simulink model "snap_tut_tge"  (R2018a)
settings: Solver=VariableStepDiscrete  StartTime=0.0  StopTime=50000  RelTol=1e-3
undefined symbols (not defined in the file): bad_frame, Bit, Both, bram, c, cnt_rst, core_rst, d, data, data_in, eof, eof_in, Falling, hex2dec, ip, ip_in, led, led_rx, led_tx, led_up, link_up, Location, Lower, Minimum_Area, notused, out, overrun, reg, Rising, ROACH2, sfp, SNAP, tx_full, tx_over, Unsigned, Upper, valid, valid_in, Width, xc7k160t
libraries: xbsIndex_r4 x1201, casper_library_misc x9, xps_library x5
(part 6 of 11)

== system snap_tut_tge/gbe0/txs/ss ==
  note: Generate stop when in circular capture mode
  note: Delay start of capture
  note: ctrl: bit0: Put a posedge here to enable a new capture. bit1: ignore external trigger and trigger immediately. bit2: ignore external write enable and capture on every FPGA clock. bit3: continuously capture data until we get an external stop command.
  note: Offset in vector from first element captured, used during circular capture
  note: Number of bytes in buffer and done bit
  note: Number of valid data samples to skip after trigger before starting capture
  note: Value on vin aligned with first sample on din captured
  din : Inport
  we : Inport  Port=2
  trig : Inport  Port=3
  add_del : xbsIndex_r4/Delay  rst=off  infoeditControl=Selection of Reset will increase slice count due to use of real FFs and instead of SRLs  en=off  latency=1  reg_retiming=on  dbl_ovrd=off  block_type=delay
  add_gen : Subsystem  AncestorBlock=casper_library_scopes/snapshot/add_gen  mask{counter_size=13+4+1, increment=16, nsamples=13, burst_size=0, use_dsp48=on}
      mask prompts: counter_size "Address counter size (2^?)"; increment "Address counter increment"; nsamples "Number of samples (2^?)"; burst_size "Burst size (2^?)"; use_dsp48 "dsp48 counter/s"
      mask init:
      | set_param(gcb,'LinkStatus','inactive');
      | if strcmp(use_dsp48,'on'),
      |     set_param([gcb,'/add_gen'],'implementation','DSP48');
      | else
      |     set_param([gcb,'/add_gen'],'implementation','Fabric');
      | end
  arm : xbsIndex_r4/Constant  const=0  gui_display_data_type=Fixed-point  arith_type=Boolean  n_bits=16  bin_pt=14  preci_type=Single  exp_width=8  frac_width=24  explicit_period=on  period=1  equ=P=C  opselect=C  inp2=PCIN>>17  opr=+  inp1=P  carry=CIN  dbl_ovrd=off  block_type=constant
  arm_or : xbsIndex_r4/Logical  logical_function=OR  inputs=2  en=off  latency=0  precision=Full  arith_type=Unsigned  n_bits=16  bin_pt=0  align_bp=on  dbl_ovrd=off  block_type=logical
  basic_ctrl : Subsystem  AncestorBlock=casper_library_scopes/snapshot/basic_ctrl  mask{dram=off, data_width=128}
      mask prompts: data_width "data width"
      mask init:
      | set_param(gcb,'LinkStatus','inactive');
      | set_param([gcb,'/dram_munge'], 'dram', dram);
  bram : Subsystem  Tag=xps:bram  AncestorBlock=xps_library/Memory/shared_bram  mask{arith_type=Unsigned, addr_width=13, data_width=128, reg_prim_output=off, reg_core_output=off, optimization=Minimum_Area, data_bin_pt=0, init_vals=[0:2^13-1], sample_rate=1}
      mask prompts: arith_type "Output Data Type"; addr_width "Address width"; data_width "Data Width"; reg_prim_output "Register Primitive Output"; reg_core_output "Register Core Output"; data_bin_pt "Data Binary Point"; init_vals "Initial values (simulation only)"; sample_rate "Sample rate"
      mask init:
      | shared_bram_mask;
  cast : xbsIndex_r4/Convert  gui_display_data_type=Fixed-point  arith_type=Unsigned  n_bits=128  bin_pt=0  float_type=Single  exp_bits=8  fraction_bits=24  quantization=Truncate  overflow=Wrap  en=off  latency=0  pipeline=off  dbl_ovrd=off  block_type=convert
  circ : xbsIndex_r4/Constant  const=0  gui_display_data_type=Fixed-point  arith_type=Boolean  n_bits=16  bin_pt=14  preci_type=Single  exp_width=8  frac_width=24  explicit_period=on  period=1  equ=P=C  opselect=C  inp2=PCIN>>17  opr=+  inp1=P  carry=CIN  dbl_ovrd=off  block_type=constant
  circ_or : xbsIndex_r4/Logical  logical_function=OR  inputs=2  en=off  latency=0  precision=Full  arith_type=Unsigned  n_bits=16  bin_pt=0  align_bp=on  dbl_ovrd=off  block_type=logical
  ctrl : Subsystem  Tag=xps:sw_reg  AncestorBlock=xps_library/Memory/software_register  mask(swreg){io_dir=From Processor, io_delay=0, init_val=0, sample_period=1, names=reg, bitwidths=32, bin_pts=0, arith_types=0, sim_port=off, show_format=on}
      mask prompts: io_dir "I/O direction"; io_delay "I/O delay"; init_val "Initial Value"; sample_period "Sample period"; names "Bitfield names [msb...lsb]"; bitwidths "Bitfield widths"; bin_pts "Bitfield binary pts"; arith_types "Bitfield types, ufix=0, fix=1, bool=2"; sim_port "Provide sim input/output?"; show_format "Print format string?"
      mask help: A 32-bit software-accessible register. Can be divided into bitfields of varying widths and types using the fields in the block mask.
      mask init:
      | swreg_init(gcb)
  ctrl_combine : Subsystem  AncestorBlock=casper_library_flow_control/bus_create  mask(bus_create){inputNum=4}
      mask prompts: inputNum "Number of inputs:"
      mask init:
      | bus_create_init(gcb,...
      |     'inputNum', inputNum);
  ctrl_split : Subsystem  AncestorBlock=casper_library_flow_control/bus_expand  mask(bus_expand){mode=divisions of arbitrary size, outputNum=1, outputWidth=[28 1 2 1], outputBinaryPt=0, outputArithmeticType=[0 2 0 2], show_format=on, outputToWorkspace=off, variablePrefix=out, outputToModelAsWell=on}
      mask prompts: outputNum "Number of outputs:"; outputWidth "Output width [msb ... lsb]:"; outputBinaryPt "Output binary point position [msb ... lsb]:"; outputArithmeticType "Output arithmetic type (ufix=0, fix=1, bool=2) [msb ... lsb]:"; show_format "Print format string?"; outputToWorkspace "Output to workspace?"; variablePrefix "Variable name prefix:"; outputToModelAsWell "Output to model as well?"
      mask help: Expands a 'bus' made using a bus_create or Xilinx concat block. The input will be divided into the specified number of outputs with the specified arithmetic types. Divisions are made from most significant bit.
      mask init:
      | bus_expand_init(gcb,...
      |     'mode', mode, ...
      |     'outputNum', outputNum, ...
      |     'outputWidth', outputWidth, ...
      |     'outputBinaryPt', outputBinaryPt, ...
      |     'outputArithmeticType', outputArithmeticType, ...
      |     'show_format', show_format, ...
      |     'outputToWorkspace', outputToWorkspace, ...
      |     'variablePrefix', variablePrefix, ...
      |     'outputToModelAsWell', outputToModelAsWell);
  dat_del : xbsIndex_r4/Delay  rst=off  infoeditControl=Selection of Reset will increase slice count due to use of real FFs and instead of SRLs  en=off  latency=1  reg_retiming=on  dbl_ovrd=off  block_type=delay
  g_tr_en_cnt : Terminator
  gbram : Terminator
  goto_ss_we2_const : xbsIndex_r4/Constant  const=0  gui_display_data_type=Fixed-point  arith_type=Boolean  n_bits=16  bin_pt=14  preci_type=Single  exp_width=8  frac_width=24  explicit_period=on  period=1  equ=P=C  opselect=C  inp2=PCIN>>17  opr=+  inp1=P  carry=CIN  dbl_ovrd=off  block_type=constant
  goto_ss_we3_const : xbsIndex_r4/Constant  const=0  gui_display_data_type=Fixed-point  arith_type=Boolean  n_bits=16  bin_pt=14  preci_type=Single  exp_width=8  frac_width=24  explicit_period=on  period=1  equ=P=C  opselect=C  inp2=PCIN>>17  opr=+  inp1=P  carry=CIN  dbl_ovrd=off  block_type=constant
  gval : Terminator
  never : xbsIndex_r4/Constant  const=0  gui_display_data_type=Fixed-point  arith_type=Boolean  n_bits=16  bin_pt=14  preci_type=Single  exp_width=8  frac_width=24  explicit_period=on  period=1  equ=P=C  opselect=C  inp2=PCIN>>17  opr=+  inp1=P  carry=CIN  dbl_ovrd=off  block_type=constant
  ri : xbsIndex_r4/Reinterpret  force_arith_type=on  arith_type=Unsigned  force_bin_pt=on  bin_pt=0  block_type=reinterpret
  status : Subsystem  Tag=xps:sw_reg  AncestorBlock=xps_library/Memory/software_register  mask(swreg){io_dir=To Processor, io_delay=0, init_val=0, sample_period=1, names=reg, bitwidths=32, bin_pts=0, arith_types=0, sim_port=off, show_format=on}
      mask prompts: io_dir "I/O direction"; io_delay "I/O delay"; init_val "Initial Value"; sample_period "Sample period"; names "Bitfield names [msb...lsb]"; bitwidths "Bitfield widths"; bin_pts "Bitfield binary pts"; arith_types "Bitfield types, ufix=0, fix=1, bool=2"; sim_port "Provide sim input/output?"; show_format "Print format string?"
      mask help: A 32-bit software-accessible register. Can be divided into bitfields of varying widths and types using the fields in the block mask.
      mask init:
      | swreg_init(gcb)
  vin_const : xbsIndex_r4/Constant  const=0  gui_display_data_type=Fixed-point  arith_type=Boolean  n_bits=16  bin_pt=14  preci_type=Single  exp_width=8  frac_width=24  explicit_period=on  period=1  equ=P=C  opselect=C  inp2=PCIN>>17  opr=+  inp1=P  carry=CIN  dbl_ovrd=off  block_type=constant
  we_del : xbsIndex_r4/Delay  rst=off  infoeditControl=Selection of Reset will increase slice count due to use of real FFs and instead of SRLs  en=off  latency=1  reg_retiming=on  dbl_ovrd=off  block_type=delay
  arm_out : Outport
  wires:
  din/1 -> ri/1
  ri/1 -> cast/1
  cast/1 -> basic_ctrl/2(din)
  we/1 -> basic_ctrl/3(we)
  trig/1 -> basic_ctrl/4(trig)
  ctrl_combine/1(bus_out) -> basic_ctrl/5(ctrl)
  never/1 -> basic_ctrl/6(stopi)
  arm/1 -> arm_or/2
  arm_or/1 -> arm_out/1, ctrl_combine/4(in4)
  circ/1 -> circ_or/2
  ctrl/1(in_reg) -> ctrl_split/1(bus_in)
  ctrl_split/1(msb_out4) -> ctrl_combine/1(in1)
  ctrl_split/2(out3) -> circ_or/1
  ctrl_split/3(out2) -> ctrl_combine/3(in3)
  ctrl_split/4(lsb_out1) -> arm_or/1
  circ_or/1 -> ctrl_combine/2(in2)
  basic_ctrl/1(vout) -> add_gen/1(vin)
  basic_ctrl/2(dout) -> add_gen/2(din)
  basic_ctrl/3(we_o) -> add_gen/3(we), [goto_80619549_we1]
  basic_ctrl/4(go) -> add_gen/4(go)
  basic_ctrl/5(stop) -> add_gen/5(cont)
  basic_ctrl/6(init) -> add_gen/6(init)
  add_gen/5(status) -> status/1(out_reg)
  vin_const/1 -> basic_ctrl/1(vin)
  add_gen/1(vout) -> gval/1
  add_gen/6(en_cnt) -> g_tr_en_cnt/1
  add_gen/2(add) -> add_del/1
  add_gen/3(dout) -> dat_del/1
  add_gen/4(we_o) -> we_del/1, [goto_80619549_we4]
  add_del/1 -> bram/1(addr)
  dat_del/1 -> bram/2(data_in)
  we_del/1 -> bram/3(we)
  bram/1(data_out) -> gbram/1
  goto_ss_we2_const/1 -> [goto_80619549_we2]
  goto_ss_we3_const/1 -> [goto_80619549_we3]

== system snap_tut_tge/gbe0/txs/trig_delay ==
  d : Inport
  Register{0..4} (5 alike) : xbsIndex_r4/Register  init=0  rst=off  en=off  dbl_ovrd=off  block_type=register
  q : Outport
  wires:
  Register0/1 -> Register1/1
  Register1/1 -> Register2/1
  Register2/1 -> Register3/1
  Register3/1 -> Register4/1
  d/1 -> Register0/1
  Register4/1 -> q/1

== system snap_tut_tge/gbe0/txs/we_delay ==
  d : Inport
  Register{0..4} (5 alike) : xbsIndex_r4/Register  init=0  rst=off  en=off  dbl_ovrd=off  block_type=register
  q : Outport
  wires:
  Register0/1 -> Register1/1
  Register1/1 -> Register2/1
  Register2/1 -> Register3/1
  Register3/1 -> Register4/1
  d/1 -> Register0/1
  Register4/1 -> q/1

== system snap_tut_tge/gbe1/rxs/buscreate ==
  in1 : Inport
  in2 : Inport  Port=2
  in3 : Inport  Port=3
  in4 : Inport  Port=4
  in5 : Inport  Port=5
  in6 : Inport  Port=6
  in7 : Inport  Port=7
  in8 : Inport  Port=8
  concatenate : xbsIndex_r4/Concat  num_inputs=8  dbl_ovrd=off  block_type=concat
  reinterpret{1..8} (8 alike) : xbsIndex_r4/Reinterpret  force_arith_type=on  arith_type=Unsigned  force_bin_pt=on  bin_pt=0  block_type=reinterpret
  bus_out : Outport
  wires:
  concatenate/1 -> bus_out/1
  in1/1 -> reinterpret1/1
  reinterpret1/1 -> concatenate/1
  in2/1 -> reinterpret2/1
  reinterpret2/1 -> concatenate/2
  in3/1 -> reinterpret3/1
  reinterpret3/1 -> concatenate/3
  in4/1 -> reinterpret4/1
  reinterpret4/1 -> concatenate/4
  in5/1 -> reinterpret5/1
  reinterpret5/1 -> concatenate/5
  in6/1 -> reinterpret6/1
  reinterpret6/1 -> concatenate/6
  in7/1 -> reinterpret7/1
  reinterpret7/1 -> concatenate/7
  in8/1 -> reinterpret8/1
  reinterpret8/1 -> concatenate/8

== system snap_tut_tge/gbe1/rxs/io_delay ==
  d : Inport
  Register{0..4} (5 alike) : xbsIndex_r4/Register  init=0  rst=off  en=off  dbl_ovrd=off  block_type=register
  q : Outport
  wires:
  Register0/1 -> Register1/1
  Register1/1 -> Register2/1
  Register2/1 -> Register3/1
  Register3/1 -> Register4/1
  d/1 -> Register0/1
  Register4/1 -> q/1

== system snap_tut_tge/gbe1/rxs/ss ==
  note: Generate stop when in circular capture mode
  note: Delay start of capture
  note: ctrl: bit0: Put a posedge here to enable a new capture. bit1: ignore external trigger and trigger immediately. bit2: ignore external write enable and capture on every FPGA clock. bit3: continuously capture data until we get an external stop command.
  note: Offset in vector from first element captured, used during circular capture
  note: Number of bytes in buffer and done bit
  note: Number of valid data samples to skip after trigger before starting capture
  note: Value on vin aligned with first sample on din captured
  din : Inport
  we : Inport  Port=2
  trig : Inport  Port=3
  add_del : xbsIndex_r4/Delay  rst=off  infoeditControl=Selection of Reset will increase slice count due to use of real FFs and instead of SRLs  en=off  latency=1  reg_retiming=on  dbl_ovrd=off  block_type=delay
  add_gen : Subsystem  AncestorBlock=casper_library_scopes/snapshot/add_gen  mask{counter_size=13+4+1, increment=16, nsamples=13, burst_size=0, use_dsp48=on}
      mask prompts: counter_size "Address counter size (2^?)"; increment "Address counter increment"; nsamples "Number of samples (2^?)"; burst_size "Burst size (2^?)"; use_dsp48 "dsp48 counter/s"
      mask init:
      | set_param(gcb,'LinkStatus','inactive');
      | if strcmp(use_dsp48,'on'),
      |     set_param([gcb,'/add_gen'],'implementation','DSP48');
      | else
      |     set_param([gcb,'/add_gen'],'implementation','Fabric');
      | end
  arm : xbsIndex_r4/Constant  const=0  gui_display_data_type=Fixed-point  arith_type=Boolean  n_bits=16  bin_pt=14  preci_type=Single  exp_width=8  frac_width=24  explicit_period=on  period=1  equ=P=C  opselect=C  inp2=PCIN>>17  opr=+  inp1=P  carry=CIN  dbl_ovrd=off  block_type=constant
  arm_or : xbsIndex_r4/Logical  logical_function=OR  inputs=2  en=off  latency=0  precision=Full  arith_type=Unsigned  n_bits=16  bin_pt=0  align_bp=on  dbl_ovrd=off  block_type=logical
  basic_ctrl : Subsystem  AncestorBlock=casper_library_scopes/snapshot/basic_ctrl  mask{dram=off, data_width=128}
      mask prompts: data_width "data width"
      mask init:
      | set_param(gcb,'LinkStatus','inactive');
      | set_param([gcb,'/dram_munge'], 'dram', dram);
  bram : Subsystem  Tag=xps:bram  AncestorBlock=xps_library/Memory/shared_bram  mask{arith_type=Unsigned, addr_width=13, data_width=128, reg_prim_output=off, reg_core_output=off, optimization=Minimum_Area, data_bin_pt=0, init_vals=[0:2^13-1], sample_rate=1}
      mask prompts: arith_type "Output Data Type"; addr_width "Address width"; data_width "Data Width"; reg_prim_output "Register Primitive Output"; reg_core_output "Register Core Output"; data_bin_pt "Data Binary Point"; init_vals "Initial values (simulation only)"; sample_rate "Sample rate"
      mask init:
      | shared_bram_mask;
  cast : xbsIndex_r4/Convert  gui_display_data_type=Fixed-point  arith_type=Unsigned  n_bits=128  bin_pt=0  float_type=Single  exp_bits=8  fraction_bits=24  quantization=Truncate  overflow=Wrap  en=off  latency=0  pipeline=off  dbl_ovrd=off  block_type=convert
  circ : xbsIndex_r4/Constant  const=0  gui_display_data_type=Fixed-point  arith_type=Boolean  n_bits=16  bin_pt=14  preci_type=Single  exp_width=8  frac_width=24  explicit_period=on  period=1  equ=P=C  opselect=C  inp2=PCIN>>17  opr=+  inp1=P  carry=CIN  dbl_ovrd=off  block_type=constant
  circ_or : xbsIndex_r4/Logical  logical_function=OR  inputs=2  en=off  latency=0  precision=Full  arith_type=Unsigned  n_bits=16  bin_pt=0  align_bp=on  dbl_ovrd=off  block_type=logical
  ctrl : Subsystem  Tag=xps:sw_reg  AncestorBlock=xps_library/Memory/software_register  mask(swreg){io_dir=From Processor, io_delay=0, init_val=0, sample_period=1, names=reg, bitwidths=32, bin_pts=0, arith_types=0, sim_port=off, show_format=on}
      mask prompts: io_dir "I/O direction"; io_delay "I/O delay"; init_val "Initial Value"; sample_period "Sample period"; names "Bitfield names [msb...lsb]"; bitwidths "Bitfield widths"; bin_pts "Bitfield binary pts"; arith_types "Bitfield types, ufix=0, fix=1, bool=2"; sim_port "Provide sim input/output?"; show_format "Print format string?"
      mask help: A 32-bit software-accessible register. Can be divided into bitfields of varying widths and types using the fields in the block mask.
      mask init:
      | swreg_init(gcb)
  ctrl_combine : Subsystem  AncestorBlock=casper_library_flow_control/bus_create  mask(bus_create){inputNum=4}
      mask prompts: inputNum "Number of inputs:"
      mask init:
      | bus_create_init(gcb,...
      |     'inputNum', inputNum);
  ctrl_split : Subsystem  AncestorBlock=casper_library_flow_control/bus_expand  mask(bus_expand){mode=divisions of arbitrary size, outputNum=1, outputWidth=[28 1 2 1], outputBinaryPt=0, outputArithmeticType=[0 2 0 2], show_format=on, outputToWorkspace=off, variablePrefix=out, outputToModelAsWell=on}
      mask prompts: outputNum "Number of outputs:"; outputWidth "Output width [msb ... lsb]:"; outputBinaryPt "Output binary point position [msb ... lsb]:"; outputArithmeticType "Output arithmetic type (ufix=0, fix=1, bool=2) [msb ... lsb]:"; show_format "Print format string?"; outputToWorkspace "Output to workspace?"; variablePrefix "Variable name prefix:"; outputToModelAsWell "Output to model as well?"
      mask help: Expands a 'bus' made using a bus_create or Xilinx concat block. The input will be divided into the specified number of outputs with the specified arithmetic types. Divisions are made from most significant bit.
      mask init:
      | bus_expand_init(gcb,...
      |     'mode', mode, ...
      |     'outputNum', outputNum, ...
      |     'outputWidth', outputWidth, ...
      |     'outputBinaryPt', outputBinaryPt, ...
      |     'outputArithmeticType', outputArithmeticType, ...
      |     'show_format', show_format, ...
      |     'outputToWorkspace', outputToWorkspace, ...
      |     'variablePrefix', variablePrefix, ...
      |     'outputToModelAsWell', outputToModelAsWell);
  dat_del : xbsIndex_r4/Delay  rst=off  infoeditControl=Selection of Reset will increase slice count due to use of real FFs and instead of SRLs  en=off  latency=1  reg_retiming=on  dbl_ovrd=off  block_type=delay
  g_tr_en_cnt : Terminator
  gbram : Terminator
  goto_ss_we2_const : xbsIndex_r4/Constant  const=0  gui_display_data_type=Fixed-point  arith_type=Boolean  n_bits=16  bin_pt=14  preci_type=Single  exp_width=8  frac_width=24  explicit_period=on  period=1  equ=P=C  opselect=C  inp2=PCIN>>17  opr=+  inp1=P  carry=CIN  dbl_ovrd=off  block_type=constant
  goto_ss_we3_const : xbsIndex_r4/Constant  const=0  gui_display_data_type=Fixed-point  arith_type=Boolean  n_bits=16  bin_pt=14  preci_type=Single  exp_width=8  frac_width=24  explicit_period=on  period=1  equ=P=C  opselect=C  inp2=PCIN>>17  opr=+  inp1=P  carry=CIN  dbl_ovrd=off  block_type=constant
  gval : Terminator
  never : xbsIndex_r4/Constant  const=0  gui_display_data_type=Fixed-point  arith_type=Boolean  n_bits=16  bin_pt=14  preci_type=Single  exp_width=8  frac_width=24  explicit_period=on  period=1  equ=P=C  opselect=C  inp2=PCIN>>17  opr=+  inp1=P  carry=CIN  dbl_ovrd=off  block_type=constant
  ri : xbsIndex_r4/Reinterpret  force_arith_type=on  arith_type=Unsigned  force_bin_pt=on  bin_pt=0  block_type=reinterpret
  status : Subsystem  Tag=xps:sw_reg  AncestorBlock=xps_library/Memory/software_register  mask(swreg){io_dir=To Processor, io_delay=0, init_val=0, sample_period=1, names=reg, bitwidths=32, bin_pts=0, arith_types=0, sim_port=off, show_format=on}
      mask prompts: io_dir "I/O direction"; io_delay "I/O delay"; init_val "Initial Value"; sample_period "Sample period"; names "Bitfield names [msb...lsb]"; bitwidths "Bitfield widths"; bin_pts "Bitfield binary pts"; arith_types "Bitfield types, ufix=0, fix=1, bool=2"; sim_port "Provide sim input/output?"; show_format "Print format string?"
      mask help: A 32-bit software-accessible register. Can be divided into bitfields of varying widths and types using the fields in the block mask.
      mask init:
      | swreg_init(gcb)
  vin_const : xbsIndex_r4/Constant  const=0  gui_display_data_type=Fixed-point  arith_type=Boolean  n_bits=16  bin_pt=14  preci_type=Single  exp_width=8  frac_width=24  explicit_period=on  period=1  equ=P=C  opselect=C  inp2=PCIN>>17  opr=+  inp1=P  carry=CIN  dbl_ovrd=off  block_type=constant
  we_del : xbsIndex_r4/Delay  rst=off  infoeditControl=Selection of Reset will increase slice count due to use of real FFs and instead of SRLs  en=off  latency=1  reg_retiming=on  dbl_ovrd=off  block_type=delay
  arm_out : Outport
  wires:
  din/1 -> ri/1
  ri/1 -> cast/1
  cast/1 -> basic_ctrl/2(din)
  we/1 -> basic_ctrl/3(we)
  trig/1 -> basic_ctrl/4(trig)
  ctrl_combine/1(bus_out) -> basic_ctrl/5(ctrl)
  never/1 -> basic_ctrl/6(stopi)
  arm/1 -> arm_or/2
  arm_or/1 -> arm_out/1, ctrl_combine/4(in4)
  circ/1 -> circ_or/2
  ctrl/1(in_reg) -> ctrl_split/1(bus_in)
  ctrl_split/1(msb_out4) -> ctrl_combine/1(in1)
  ctrl_split/2(out3) -> circ_or/1
  ctrl_split/3(out2) -> ctrl_combine/3(in3)
  ctrl_split/4(lsb_out1) -> arm_or/1
  circ_or/1 -> ctrl_combine/2(in2)
  basic_ctrl/1(vout) -> add_gen/1(vin)
  basic_ctrl/2(dout) -> add_gen/2(din)
  basic_ctrl/3(we_o) -> add_gen/3(we), [goto_21341118_we1]
  basic_ctrl/4(go) -> add_gen/4(go)
  basic_ctrl/5(stop) -> add_gen/5(cont)
  basic_ctrl/6(init) -> add_gen/6(init)
  add_gen/5(status) -> status/1(out_reg)
  vin_const/1 -> basic_ctrl/1(vin)
  add_gen/1(vout) -> gval/1
  add_gen/6(en_cnt) -> g_tr_en_cnt/1
  add_gen/2(add) -> add_del/1
  add_gen/3(dout) -> dat_del/1
  add_gen/4(we_o) -> we_del/1, [goto_21341118_we4]
  add_del/1 -> bram/1(addr)
  dat_del/1 -> bram/2(data_in)
  we_del/1 -> bram/3(we)
  bram/1(data_out) -> gbram/1
  goto_ss_we2_const/1 -> [goto_21341118_we2]
  goto_ss_we3_const/1 -> [goto_21341118_we3]

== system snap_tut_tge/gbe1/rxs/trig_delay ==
  d : Inport
  Register{0..4} (5 alike) : xbsIndex_r4/Register  init=0  rst=off  en=off  dbl_ovrd=off  block_type=register
  q : Outport
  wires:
  Register0/1 -> Register1/1
  Register1/1 -> Register2/1
  Register2/1 -> Register3/1
  Register3/1 -> Register4/1
  d/1 -> Register0/1
  Register4/1 -> q/1

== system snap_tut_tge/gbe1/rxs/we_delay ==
  d : Inport
  Register{0..4} (5 alike) : xbsIndex_r4/Register  init=0  rst=off  en=off  dbl_ovrd=off  block_type=register
  q : Outport
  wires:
  Register0/1 -> Register1/1
  Register1/1 -> Register2/1
  Register2/1 -> Register3/1
  Register3/1 -> Register4/1
  d/1 -> Register0/1
  Register4/1 -> q/1

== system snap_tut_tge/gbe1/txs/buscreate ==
  in1 : Inport
  in2 : Inport  Port=2
  in3 : Inport  Port=3
  in4 : Inport  Port=4
  in5 : Inport  Port=5
  in6 : Inport  Port=6
  in7 : Inport  Port=7
  in8 : Inport  Port=8
  concatenate : xbsIndex_r4/Concat  num_inputs=8  dbl_ovrd=off  block_type=concat
  reinterpret{1..8} (8 alike) : xbsIndex_r4/Reinterpret  force_arith_type=on  arith_type=Unsigned  force_bin_pt=on  bin_pt=0  block_type=reinterpret
  bus_out : Outport
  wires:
  concatenate/1 -> bus_out/1
  in1/1 -> reinterpret1/1
  reinterpret1/1 -> concatenate/1
  in2/1 -> reinterpret2/1
  reinterpret2/1 -> concatenate/2
  in3/1 -> reinterpret3/1
  reinterpret3/1 -> concatenate/3
  in4/1 -> reinterpret4/1
  reinterpret4/1 -> concatenate/4
  in5/1 -> reinterpret5/1
  reinterpret5/1 -> concatenate/5
  in6/1 -> reinterpret6/1
  reinterpret6/1 -> concatenate/6
  in7/1 -> reinterpret7/1
  reinterpret7/1 -> concatenate/7
  in8/1 -> reinterpret8/1
  reinterpret8/1 -> concatenate/8

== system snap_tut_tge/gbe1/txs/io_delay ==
  d : Inport
  Register{0..4} (5 alike) : xbsIndex_r4/Register  init=0  rst=off  en=off  dbl_ovrd=off  block_type=register
  q : Outport
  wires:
  Register0/1 -> Register1/1
  Register1/1 -> Register2/1
  Register2/1 -> Register3/1
  Register3/1 -> Register4/1
  d/1 -> Register0/1
  Register4/1 -> q/1

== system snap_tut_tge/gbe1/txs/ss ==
  note: Generate stop when in circular capture mode
  note: Delay start of capture
  note: ctrl: bit0: Put a posedge here to enable a new capture. bit1: ignore external trigger and trigger immediately. bit2: ignore external write enable and capture on every FPGA clock. bit3: continuously capture data until we get an external stop command.
  note: Offset in vector from first element captured, used during circular capture
  note: Number of bytes in buffer and done bit
  note: Number of valid data samples to skip after trigger before starting capture
  note: Value on vin aligned with first sample on din captured
  din : Inport
  we : Inport  Port=2
  trig : Inport  Port=3
  add_del : xbsIndex_r4/Delay  rst=off  infoeditControl=Selection of Reset will increase slice count due to use of real FFs and instead of SRLs  en=off  latency=1  reg_retiming=on  dbl_ovrd=off  block_type=delay
  add_gen : Subsystem  AncestorBlock=casper_library_scopes/snapshot/add_gen  mask{counter_size=13+4+1, increment=16, nsamples=13, burst_size=0, use_dsp48=on}
      mask prompts: counter_size "Address counter size (2^?)"; increment "Address counter increment"; nsamples "Number of samples (2^?)"; burst_size "Burst size (2^?)"; use_dsp48 "dsp48 counter/s"
      mask init:
      | set_param(gcb,'LinkStatus','inactive');
      | if strcmp(use_dsp48,'on'),
      |     set_param([gcb,'/add_gen'],'implementation','DSP48');
      | else
      |     set_param([gcb,'/add_gen'],'implementation','Fabric');
      | end
  arm : xbsIndex_r4/Constant  const=0  gui_display_data_type=Fixed-point  arith_type=Boolean  n_bits=16  bin_pt=14  preci_type=Single  exp_width=8  frac_width=24  explicit_period=on  period=1  equ=P=C  opselect=C  inp2=PCIN>>17  opr=+  inp1=P  carry=CIN  dbl_ovrd=off  block_type=constant
  arm_or : xbsIndex_r4/Logical  logical_function=OR  inputs=2  en=off  latency=0  precision=Full  arith_type=Unsigned  n_bits=16  bin_pt=0  align_bp=on  dbl_ovrd=off  block_type=logical
  basic_ctrl : Subsystem  AncestorBlock=casper_library_scopes/snapshot/basic_ctrl  mask{dram=off, data_width=128}
      mask prompts: data_width "data width"
      mask init:
      | set_param(gcb,'LinkStatus','inactive');
      | set_param([gcb,'/dram_munge'], 'dram', dram);
  bram : Subsystem  Tag=xps:bram  AncestorBlock=xps_library/Memory/shared_bram  mask{arith_type=Unsigned, addr_width=13, data_width=128, reg_prim_output=off, reg_core_output=off, optimization=Minimum_Area, data_bin_pt=0, init_vals=[0:2^13-1], sample_rate=1}
      mask prompts: arith_type "Output Data Type"; addr_width "Address width"; data_width "Data Width"; reg_prim_output "Register Primitive Output"; reg_core_output "Register Core Output"; data_bin_pt "Data Binary Point"; init_vals "Initial values (simulation only)"; sample_rate "Sample rate"
      mask init:
      | shared_bram_mask;
  cast : xbsIndex_r4/Convert  gui_display_data_type=Fixed-point  arith_type=Unsigned  n_bits=128  bin_pt=0  float_type=Single  exp_bits=8  fraction_bits=24  quantization=Truncate  overflow=Wrap  en=off  latency=0  pipeline=off  dbl_ovrd=off  block_type=convert
  circ : xbsIndex_r4/Constant  const=0  gui_display_data_type=Fixed-point  arith_type=Boolean  n_bits=16  bin_pt=14  preci_type=Single  exp_width=8  frac_width=24  explicit_period=on  period=1  equ=P=C  opselect=C  inp2=PCIN>>17  opr=+  inp1=P  carry=CIN  dbl_ovrd=off  block_type=constant
  circ_or : xbsIndex_r4/Logical  logical_function=OR  inputs=2  en=off  latency=0  precision=Full  arith_type=Unsigned  n_bits=16  bin_pt=0  align_bp=on  dbl_ovrd=off  block_type=logical
  ctrl : Subsystem  Tag=xps:sw_reg  AncestorBlock=xps_library/Memory/software_register  mask(swreg){io_dir=From Processor, io_delay=0, init_val=0, sample_period=1, names=reg, bitwidths=32, bin_pts=0, arith_types=0, sim_port=off, show_format=on}
      mask prompts: io_dir "I/O direction"; io_delay "I/O delay"; init_val "Initial Value"; sample_period "Sample period"; names "Bitfield names [msb...lsb]"; bitwidths "Bitfield widths"; bin_pts "Bitfield binary pts"; arith_types "Bitfield types, ufix=0, fix=1, bool=2"; sim_port "Provide sim input/output?"; show_format "Print format string?"
      mask help: A 32-bit software-accessible register. Can be divided into bitfields of varying widths and types using the fields in the block mask.
      mask init:
      | swreg_init(gcb)
  ctrl_combine : Subsystem  AncestorBlock=casper_library_flow_control/bus_create  mask(bus_create){inputNum=4}
      mask prompts: inputNum "Number of inputs:"
      mask init:
      | bus_create_init(gcb,...
      |     'inputNum', inputNum);
  ctrl_split : Subsystem  AncestorBlock=casper_library_flow_control/bus_expand  mask(bus_expand){mode=divisions of arbitrary size, outputNum=1, outputWidth=[28 1 2 1], outputBinaryPt=0, outputArithmeticType=[0 2 0 2], show_format=on, outputToWorkspace=off, variablePrefix=out, outputToModelAsWell=on}
      mask prompts: outputNum "Number of outputs:"; outputWidth "Output width [msb ... lsb]:"; outputBinaryPt "Output binary point position [msb ... lsb]:"; outputArithmeticType "Output arithmetic type (ufix=0, fix=1, bool=2) [msb ... lsb]:"; show_format "Print format string?"; outputToWorkspace "Output to workspace?"; variablePrefix "Variable name prefix:"; outputToModelAsWell "Output to model as well?"
      mask help: Expands a 'bus' made using a bus_create or Xilinx concat block. The input will be divided into the specified number of outputs with the specified arithmetic types. Divisions are made from most significant bit.
      mask init:
      | bus_expand_init(gcb,...
      |     'mode', mode, ...
      |     'outputNum', outputNum, ...
      |     'outputWidth', outputWidth, ...
      |     'outputBinaryPt', outputBinaryPt, ...
      |     'outputArithmeticType', outputArithmeticType, ...
      |     'show_format', show_format, ...
      |     'outputToWorkspace', outputToWorkspace, ...
      |     'variablePrefix', variablePrefix, ...
      |     'outputToModelAsWell', outputToModelAsWell);
  dat_del : xbsIndex_r4/Delay  rst=off  infoeditControl=Selection of Reset will increase slice count due to use of real FFs and instead of SRLs  en=off  latency=1  reg_retiming=on  dbl_ovrd=off  block_type=delay
  g_tr_en_cnt : Terminator
  gbram : Terminator
  goto_ss_we2_const : xbsIndex_r4/Constant  const=0  gui_display_data_type=Fixed-point  arith_type=Boolean  n_bits=16  bin_pt=14  preci_type=Single  exp_width=8  frac_width=24  explicit_period=on  period=1  equ=P=C  opselect=C  inp2=PCIN>>17  opr=+  inp1=P  carry=CIN  dbl_ovrd=off  block_type=constant
  goto_ss_we3_const : xbsIndex_r4/Constant  const=0  gui_display_data_type=Fixed-point  arith_type=Boolean  n_bits=16  bin_pt=14  preci_type=Single  exp_width=8  frac_width=24  explicit_period=on  period=1  equ=P=C  opselect=C  inp2=PCIN>>17  opr=+  inp1=P  carry=CIN  dbl_ovrd=off  block_type=constant
  gval : Terminator
  never : xbsIndex_r4/Constant  const=0  gui_display_data_type=Fixed-point  arith_type=Boolean  n_bits=16  bin_pt=14  preci_type=Single  exp_width=8  frac_width=24  explicit_period=on  period=1  equ=P=C  opselect=C  inp2=PCIN>>17  opr=+  inp1=P  carry=CIN  dbl_ovrd=off  block_type=constant
  ri : xbsIndex_r4/Reinterpret  force_arith_type=on  arith_type=Unsigned  force_bin_pt=on  bin_pt=0  block_type=reinterpret
  status : Subsystem  Tag=xps:sw_reg  AncestorBlock=xps_library/Memory/software_register  mask(swreg){io_dir=To Processor, io_delay=0, init_val=0, sample_period=1, names=reg, bitwidths=32, bin_pts=0, arith_types=0, sim_port=off, show_format=on}
      mask prompts: io_dir "I/O direction"; io_delay "I/O delay"; init_val "Initial Value"; sample_period "Sample period"; names "Bitfield names [msb...lsb]"; bitwidths "Bitfield widths"; bin_pts "Bitfield binary pts"; arith_types "Bitfield types, ufix=0, fix=1, bool=2"; sim_port "Provide sim input/output?"; show_format "Print format string?"
      mask help: A 32-bit software-accessible register. Can be divided into bitfields of varying widths and types using the fields in the block mask.
      mask init:
      | swreg_init(gcb)
  vin_const : xbsIndex_r4/Constant  const=0  gui_display_data_type=Fixed-point  arith_type=Boolean  n_bits=16  bin_pt=14  preci_type=Single  exp_width=8  frac_width=24  explicit_period=on  period=1  equ=P=C  opselect=C  inp2=PCIN>>17  opr=+  inp1=P  carry=CIN  dbl_ovrd=off  block_type=constant
  we_del : xbsIndex_r4/Delay  rst=off  infoeditControl=Selection of Reset will increase slice count due to use of real FFs and instead of SRLs  en=off  latency=1  reg_retiming=on  dbl_ovrd=off  block_type=delay
  arm_out : Outport
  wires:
  din/1 -> ri/1
  ri/1 -> cast/1
  cast/1 -> basic_ctrl/2(din)
  we/1 -> basic_ctrl/3(we)
  trig/1 -> basic_ctrl/4(trig)
  ctrl_combine/1(bus_out) -> basic_ctrl/5(ctrl)
  never/1 -> basic_ctrl/6(stopi)
  arm/1 -> arm_or/2
  arm_or/1 -> arm_out/1, ctrl_combine/4(in4)
  circ/1 -> circ_or/2
  ctrl/1(in_reg) -> ctrl_split/1(bus_in)
  ctrl_split/1(msb_out4) -> ctrl_combine/1(in1)
  ctrl_split/2(out3) -> circ_or/1
  ctrl_split/3(out2) -> ctrl_combine/3(in3)
  ctrl_split/4(lsb_out1) -> arm_or/1
  circ_or/1 -> ctrl_combine/2(in2)
  basic_ctrl/1(vout) -> add_gen/1(vin)
  basic_ctrl/2(dout) -> add_gen/2(din)
  basic_ctrl/3(we_o) -> add_gen/3(we), [goto_78599420_we1]
  basic_ctrl/4(go) -> add_gen/4(go)
  basic_ctrl/5(stop) -> add_gen/5(cont)
  basic_ctrl/6(init) -> add_gen/6(init)
  add_gen/5(status) -> status/1(out_reg)
  vin_const/1 -> basic_ctrl/1(vin)
  add_gen/1(vout) -> gval/1
  add_gen/6(en_cnt) -> g_tr_en_cnt/1
  add_gen/2(add) -> add_del/1
  add_gen/3(dout) -> dat_del/1
  add_gen/4(we_o) -> we_del/1, [goto_78599420_we4]
  add_del/1 -> bram/1(addr)
  dat_del/1 -> bram/2(data_in)
  we_del/1 -> bram/3(we)
  bram/1(data_out) -> gbram/1
  goto_ss_we2_const/1 -> [goto_78599420_we2]
  goto_ss_we3_const/1 -> [goto_78599420_we3]

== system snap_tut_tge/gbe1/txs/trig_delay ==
  d : Inport
  Register{0..4} (5 alike) : xbsIndex_r4/Register  init=0  rst=off  en=off  dbl_ovrd=off  block_type=register
  q : Outport
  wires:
  Register0/1 -> Register1/1
  Register1/1 -> Register2/1
  Register2/1 -> Register3/1
  Register3/1 -> Register4/1
  d/1 -> Register0/1
  Register4/1 -> q/1

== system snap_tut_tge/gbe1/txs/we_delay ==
  d : Inport
  Register{0..4} (5 alike) : xbsIndex_r4/Register  init=0  rst=off  en=off  dbl_ovrd=off  block_type=register
  q : Outport
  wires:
  Register0/1 -> Register1/1
  Register1/1 -> Register2/1
  Register2/1 -> Register3/1
  Register3/1 -> Register4/1
  d/1 -> Register0/1
  Register4/1 -> q/1

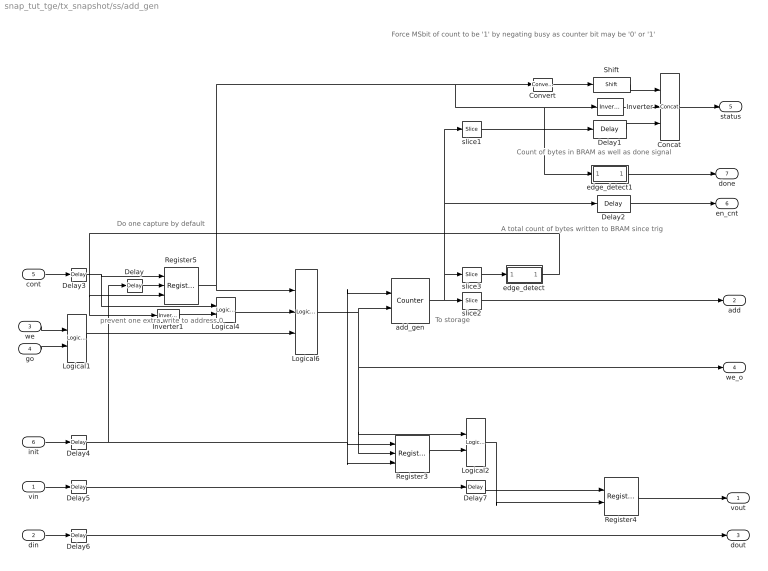
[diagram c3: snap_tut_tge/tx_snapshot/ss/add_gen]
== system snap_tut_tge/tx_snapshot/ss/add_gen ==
  note: Force MSbit of count to be '1' by negating busy as counter bit may be '0' or '1'
  note: A total count of bytes written to BRAM since trig
  note: Count of bytes in BRAM as well as done signal
  note: Do one capture by default
  note: prevent one extra write to address 0
  note: To storage
  vin : Inport
  din : Inport  Port=2
  we : Inport  Port=3
  go : Inport  Port=4
  cont : Inport  Port=5
  init : Inport  Port=6
  Concat : xbsIndex_r4/Concat  num_inputs=3  dbl_ovrd=off  block_type=concat
  Convert : xbsIndex_r4/Convert  gui_display_data_type=Fixed-point  arith_type=Unsigned  n_bits=32-nsamples-log2(increment)-1  bin_pt=0  float_type=Single  exp_bits=8  fraction_bits=24  quantization=Truncate  overflow=Wrap  en=off  latency=0  pipeline=off  dbl_ovrd=off  block_type=convert
  Delay{,3..6} (5 alike) : xbsIndex_r4/Delay  rst=off  infoeditControl=Selection of Reset will increase slice count due to use of real FFs and instead of SRLs  en=off  latency=1  reg_retiming=on  dbl_ovrd=off  block_type=delay
  Delay1 : xbsIndex_r4/Delay  rst=off  infoeditControl=Selection of Reset will increase slice count due to use of real FFs and instead of SRLs  en=off  latency=1  reg_retiming=off  dbl_ovrd=off  block_type=delay
  Delay2 : xbsIndex_r4/Delay  rst=off  infoeditControl=Selection of Reset will increase slice count due to use of real FFs and instead of SRLs  en=off  latency=1  reg_retiming=off  dbl_ovrd=off  block_type=delay
  Delay7 : xbsIndex_r4/Delay  rst=off  infoeditControl=Selection of Reset will increase slice count due to use of real FFs and instead of SRLs  en=off  latency=1  reg_retiming=off  dbl_ovrd=off  block_type=delay
  Inverter : xbsIndex_r4/Inverter  en=off  latency=1  dbl_ovrd=off  block_type=inv
  Inverter1 : xbsIndex_r4/Inverter  en=off  latency=0  dbl_ovrd=off  block_type=inv
  Logical1 : xbsIndex_r4/Logical  logical_function=AND  inputs=2  en=off  latency=1  precision=Full  arith_type=Unsigned  n_bits=8  bin_pt=2  align_bp=on  dbl_ovrd=off  block_type=logical
  Logical2 : xbsIndex_r4/Logical  logical_function=AND  inputs=2  en=off  latency=1  precision=Full  arith_type=Unsigned  n_bits=8  bin_pt=2  align_bp=on  dbl_ovrd=off  block_type=logical
  Logical4 : xbsIndex_r4/Logical  logical_function=OR  inputs=2  en=off  latency=0  precision=Full  arith_type=Unsigned  n_bits=8  bin_pt=2  align_bp=on  dbl_ovrd=off  block_type=logical
  Logical6 : xbsIndex_r4/Logical  logical_function=AND  inputs=3  en=off  latency=0  precision=Full  arith_type=Unsigned  n_bits=8  bin_pt=2  align_bp=on  dbl_ovrd=off  block_type=logical
  Register3 : xbsIndex_r4/Register  init=0  rst=on  en=on  dbl_ovrd=off  block_type=register
  Register4 : xbsIndex_r4/Register  init=0  rst=off  en=on  dbl_ovrd=off  block_type=register
  Register5 : xbsIndex_r4/Register  init=1  rst=on  en=on  dbl_ovrd=off  block_type=register
  Shift : xbsIndex_r4/Shift  shift_dir=Left  shift_bits=32-nsamples-log2(increment)-1-1  en=off  latency=1  precision=Full  arith_type="Signed  (2's comp)"  n_bits=16  bin_pt=14  quantization=Truncate  overflow=Wrap  dbl_ovrd=off  block_type=shift
  add_gen : xbsIndex_r4/Counter  cnt_type=Free Running  cnt_to=1  operation=Up  start_count=0  cnt_by_val=increment  arith_type=Unsigned  n_bits=counter_size  bin_pt=0  load_pin=off  rst=on  en=on  explicit_period=on  period=1  use_behavioral_HDL=off  implementation=DSP48  use_rpm=on  dbl_ovrd=off  block_type=counter
  edge_detect : Subsystem  AncestorBlock=casper_library_misc/edge_detect  mask(edge_detect){edge=Both, polarity=Active High, x_in=[0 0.08 0.08 0.16 0.16 0.24 0.24 0.32 0.32 0.4], y_in=[-1 -1  1  1  1  1 -1 -1 -1 -1], x_out=[0.6 0.68 0.68 0.76 0.76 0.84 0.84 0.92 0.92 1], y_out=[-1 -1  1  1 -1 -1  1  1 -1 -1]}
      mask prompts: edge "Edge Type"; polarity "Output Polarity"; x_in "Input X Positions"; y_in "Input Y Positions"; x_out "Output X Positions"; y_out "Output Y Positions"
      mask help: Output is active for one-cycle after each edge of the specified type (i.e. rising, falling or both).
      mask init:
      | edge_detect_init(gcb,...
      |     'edge',edge,...
      |     'polarity',polarity,...
      |     'x_in',x_in,...
      |     'x_out',x_out,...
      |     'y_in',y_in,...
      |     'y_out',y_out);
      | 
      | x_in_num=str2num(getfield(getfield(get_param(gcb,'UserData'),'parameters'),'x_in'));
      | x_out_num=str2num(getfield(getfield(get_param(gcb,'UserData'),'parameters'),'x_out'));
      | y_in_num=str2num(getfield(getfield(get_param(gcb,'UserData'),'parameters'),'y_in'));
      | y_out_num=str2num(getfield(getfield(get_param(gcb,'UserData'),'parameters'),'y_out'));
  edge_detect1 : Subsystem  AncestorBlock=casper_library_scopes/snapshot/add_gen/edge_detect  mask(edge_detect){edge=Both, polarity=Active High, x_in=[0 0.08 0.08 0.16 0.16 0.24 0.24 0.32 0.32 0.4], y_in=[-1 -1  1  1  1  1 -1 -1 -1 -1], x_out=[0.6 0.68 0.68 0.76 0.76 0.84 0.84 0.92 0.92 1], y_out=[-1 -1  1  1 -1 -1  1  1 -1 -1]}
      mask prompts: edge "Edge Type"; polarity "Output Polarity"; x_in "Input X Positions"; y_in "Input Y Positions"; x_out "Output X Positions"; y_out "Output Y Positions"
      mask help: Output is active for one-cycle after each edge of the specified type (i.e. rising, falling or both).
      mask init:
      | edge_detect_init(gcb,...
      |     'edge',edge,...
      |     'polarity',polarity,...
      |     'x_in',x_in,...
      |     'x_out',x_out,...
      |     'y_in',y_in,...
      |     'y_out',y_out);
      | 
      | x_in_num=str2num(getfield(getfield(get_param(gcb,'UserData'),'parameters'),'x_in'));
      | x_out_num=str2num(getfield(getfield(get_param(gcb,'UserData'),'parameters'),'x_out'));
      | y_in_num=str2num(getfield(getfield(get_param(gcb,'UserData'),'parameters'),'y_in'));
      | y_out_num=str2num(getfield(getfield(get_param(gcb,'UserData'),'parameters'),'y_out'));
  slice1 : xbsIndex_r4/Slice  nbits=nsamples+log2(increment)  boolean_output=off  mode=Lower Bit Location + Width  bit1=0  base1=LSB of Input  bit0=0  base0=LSB of Input  dbl_ovrd=off  block_type=slice
  slice2 : xbsIndex_r4/Slice  nbits=nsamples-burst_size  boolean_output=off  mode=Lower Bit Location + Width  bit1=0  base1=LSB of Input  bit0=log2(increment)+burst_size  base0=LSB of Input  dbl_ovrd=off  block_type=slice
  slice3 : xbsIndex_r4/Slice  nbits=1  boolean_output=on  mode=Lower Bit Location + Width  bit1=0  base1=MSB of Input  bit0=nsamples + log2(increment)  base0=LSB of Input  dbl_ovrd=off  block_type=slice
  vout : Outport
  add : Outport  Port=2
  dout : Outport  Port=3
  we_o : Outport  Port=4
  status : Outport  Port=5
  en_cnt : Outport  Port=6
  done : Outport  Port=7
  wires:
  Delay6/1 -> dout/1
  Delay5/1 -> Delay7/1
  Delay4/1 -> Delay/1, Register3/1, Register3/3, add_gen/1
  Delay3/1 -> Register5/1, Logical4/1
  Delay7/1 -> Register4/1
  Logical1/1 -> Logical6/3
  go/1 -> Logical1/2
  we/1 -> Logical1/1
  Logical4/1 -> Logical6/2
  Inverter/1 -> Concat/2
  slice1/1 -> Delay1/1
  Delay1/1 -> Concat/3
  din/1 -> Delay6/1
  Delay2/1 -> en_cnt/1
  slice2/1 -> add/1
  Convert/1 -> Shift/1
  Concat/1 -> status/1
  Logical6/1 -> add_gen/2, Register3/2, Logical2/1, we_o/1
  init/1 -> Delay4/1
  slice3/1 -> edge_detect/1(in)
  Register5/1 -> Logical6/1, edge_detect1/1(in), Inverter/1, Convert/1
  add_gen/1 -> slice3/1, Delay2/1, slice1/1, slice2/1
  vin/1 -> Delay5/1
  Register3/1 -> Logical2/2
  Logical2/1 -> Register4/2
  Register4/1 -> vout/1
  edge_detect/1(out) -> Register5/3, Inverter1/1
  cont/1 -> Delay3/1
  Inverter1/1 -> Logical4/2
  Delay/1 -> Register5/2
  Shift/1 -> Concat/1
  edge_detect1/1(out) -> done/1

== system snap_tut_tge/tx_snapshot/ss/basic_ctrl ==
  vin : Inport
  din : Inport  Port=2
  we : Inport  Port=3
  trig : Inport  Port=4
  ctrl : Inport  Port=5
  stopi : Inport  Port=6
  Constant : xbsIndex_r4/Constant  const=1  gui_display_data_type=Fixed-point  arith_type=Boolean  n_bits=16  bin_pt=14  preci_type=Single  exp_width=8  frac_width=24  explicit_period=on  period=1  equ=P=C  opselect=C  inp2=PCIN>>17  opr=+  inp1=P  carry=CIN  dbl_ovrd=off  block_type=constant
  Constant1 : xbsIndex_r4/Constant  const=1  gui_display_data_type=Fixed-point  arith_type=Boolean  n_bits=1  bin_pt=0  preci_type=Single  exp_width=8  frac_width=24  explicit_period=on  period=1  equ=P=C  opselect=C  inp2=PCIN>>17  opr=+  inp1=P  carry=CIN  dbl_ovrd=off  block_type=constant
  Constant2 : xbsIndex_r4/Constant  const=1  gui_display_data_type=Fixed-point  arith_type=Boolean  n_bits=1  bin_pt=0  preci_type=Single  exp_width=8  frac_width=24  explicit_period=on  period=1  equ=P=C  opselect=C  inp2=PCIN>>17  opr=+  inp1=P  carry=CIN  dbl_ovrd=off  block_type=constant
  Delay1 : xbsIndex_r4/Delay  rst=off  infoeditControl=Selection of Reset will increase slice count due to use of real FFs and instead of SRLs  en=off  latency=1  reg_retiming=off  dbl_ovrd=off  block_type=delay
  Delay2 : xbsIndex_r4/Delay  rst=off  infoeditControl=Selection of Reset will increase slice count due to use of real FFs and instead of SRLs  en=off  latency=1  reg_retiming=off  dbl_ovrd=off  block_type=delay
  Delay3 : xbsIndex_r4/Delay  rst=off  infoeditControl=Selection of Reset will increase slice count due to use of real FFs and instead of SRLs  en=off  latency=1  reg_retiming=off  dbl_ovrd=off  block_type=delay
  Inverter : xbsIndex_r4/Inverter  en=off  latency=0  dbl_ovrd=off  block_type=inv
  Logical : xbsIndex_r4/Logical  logical_function=AND  inputs=2  en=off  latency=0  precision=Full  arith_type=Unsigned  n_bits=16  bin_pt=0  align_bp=on  dbl_ovrd=off  block_type=logical
  Mux1 : xbsIndex_r4/Mux  inputs=2  en=off  latency=0  precision=Full  arith_type="Signed  (2's comp)"  n_bits=8  bin_pt=2  quantization=Truncate  overflow=Wrap  dbl_ovrd=off  block_type=mux
  Mux2 : xbsIndex_r4/Mux  inputs=2  en=off  latency=0  precision=Full  arith_type="Signed  (2's comp)"  n_bits=8  bin_pt=2  quantization=Truncate  overflow=Wrap  dbl_ovrd=off  block_type=mux
  Register1 : xbsIndex_r4/Register  init=0  rst=on  en=on  dbl_ovrd=off  block_type=register
  Register6 : xbsIndex_r4/Register  init=0  rst=on  en=on  dbl_ovrd=off  block_type=register
  dram_munge : Subsystem  mask{dram=off, data_width=data_width}
      mask prompts: data_width "data width"
      mask init:
      | set_param(gcb,'LinkStatus','inactive');
      | if strcmp(dram,'on'),
      |     set_param([gcb,'/dram'], 'const', '1');
      | else,
      |     set_param([gcb,'/dram'], 'const', '0');
      | end
      | set_param([gcb,'/data_choice'], ...
      |         'precision', 'User Defined', ...
      |         'arith_type', 'Unsigned', ...
      |         'n_bits', num2str(data_width), 'bin_pt', '0', ...
      |         'quantization', 'Truncate', ...
      |         'overflow', 'Wrap');
  edge_detect : casper_library_misc/edge_detect  edge=Rising  polarity=Active High  x_in=[0 0.08 0.08 0.16 0.16 0.24 0.24 0.32 0.32 0.4]  y_in="[-1 -1  1  1  1  1  1  1  1  1]"  x_out=[0.6 0.68 0.68 0.76 0.76 0.84 0.84 0.92 0.92 1]  y_out="[-1 -1  1  1 -1 -1 -1 -1 -1 -1]"
      link override Delay: sg_icon_stat=45,16,1,1,white,blue,0,07b98262,right,,[ ],[ ]  sg_mask_display=fprintf('','COMMENT: begin icon graphics'); patch([0 45 45 0 0 ],[0 0 16 16 0 ],[0.77 0.82 0.91 ]); plot([0 45 45 0 0 ],[0 0 16 16 0 ]); patch([17.55 20.44 22.44 24.44 26.44 22.44 19.55 17.55 ],[10.22 10.22 12.22 10.22 12.22 12.22 12.22 10.22 ],[1 1 1 ]); patch([19.55 22.44 20.44 17.55 19.55 ],[8.22 8.22 10.22 10.22 8.22 ],[0.931 0.946 0.973 ]); patch([17.55 20.44 22.44 19.55 17.55 ],[6.22 6.22 8.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
      link override Inverter: sg_icon_stat=45,16,1,1,white,blue,0,267846e5,right,,[ ],[ ]  sg_mask_display=fprintf('','COMMENT: begin icon graphics'); patch([0 45 45 0 0 ],[0 0 16 16 0 ],[0.77 0.82 0.91 ]); plot([0 45 45 0 0 ],[0 0 16 16 0 ]); patch([17.55 20.44 22.44 24.44 26.44 22.44 19.55 17.55 ],[10.22 10.22 12.22 10.22 12.22 12.22 12.22 10.22 ],[1 1 1 ]); patch([19.55 22.44 20.44 17.55 19.55 ],[8.22 8.22 10.22 10.22 8.22 ],[0.931 0.946 0.973 ]); patch([17.55 20.44 22.44 19.55 17.55 ],[6.22 6.22 8.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
      link override edge_op: sg_icon_stat=45,44,2,1,white,blue,0,affe8783,right,,[ ],[ ]  sg_mask_display=fprintf('','COMMENT: begin icon graphics'); patch([0 45 45 0 0 ],[0 0 44 44 0 ],[0.77 0.82 0.91 ]); plot([0 45 45 0 0 ],[0 0 44 44 0 ]); patch([8.65 17.32 23.32 29.32 35.32 23.32 14.65 8.65 ],[28.66 28.66 34.66 28.66 34.66 34.66 34.66 28.66 ],[1 1 1 ]); patch([14.65 23.32 17.32 8.65 14.65 ],[22.66 22.66 28.66 28.66 22.66 ],[0.931 0.946 0.973 ]); patch([8.65 17.32 23.32 14.65 8.65 ],[16.66 16.66 22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
  enable : xbsIndex_r4/Slice  nbits=1  boolean_output=on  mode=Lower Bit Location + Width  bit1=0  base1=LSB of Input  bit0=0  base0=LSB of Input  dbl_ovrd=off  block_type=slice
  trig_src : xbsIndex_r4/Slice  nbits=1  boolean_output=on  mode=Lower Bit Location + Width  bit1=0  base1=LSB of Input  bit0=1  base0=LSB of Input  dbl_ovrd=off  block_type=slice
  valid_src : xbsIndex_r4/Slice  nbits=1  boolean_output=on  mode=Lower Bit Location + Width  bit1=0  base1=LSB of Input  bit0=2  base0=LSB of Input  dbl_ovrd=off  block_type=slice
  vout : Outport
  dout : Outport  Port=2
  we_o : Outport  Port=3
  go : Outport  Port=4
  stop : Outport  Port=5
  init : Outport  Port=6
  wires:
  Delay1/1 -> edge_detect/1
  Delay3/1 -> Mux1/1
  Delay2/1 -> Mux2/1
  dram_munge/1(vout) -> vout/1
  vin/1 -> dram_munge/1(vin)
  dram_munge/3(we_o) -> we_o/1
  dram_munge/2(dout) -> dout/1
  din/1 -> dram_munge/2(din)
  Inverter/1 -> Logical/2
  Mux2/1 -> Logical/1, Register6/1
  Register6/1 -> go/1
  trig/1 -> Mux2/2
  Mux1/1 -> dram_munge/3(we)
  we/1 -> Mux1/2
  ctrl/1 -> enable/1, valid_src/1, trig_src/1
  edge_detect/1 -> Inverter/1, Register1/3, dram_munge/4(init), Register6/2, init/1
  enable/1 -> Delay1/1
  Constant1/1 -> Mux2/3
  Constant2/1 -> Mux1/3
  trig_src/1 -> Delay2/1
  valid_src/1 -> Delay3/1
  Constant/1 -> Register1/1
  Register1/1 -> Register6/3
  Logical/1 -> Register1/2
  stopi/1 -> stop/1
